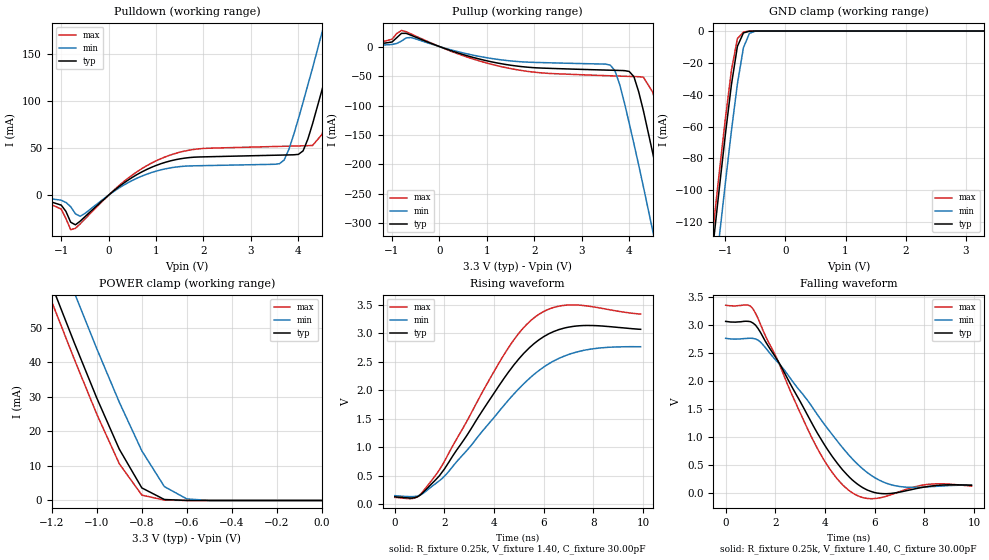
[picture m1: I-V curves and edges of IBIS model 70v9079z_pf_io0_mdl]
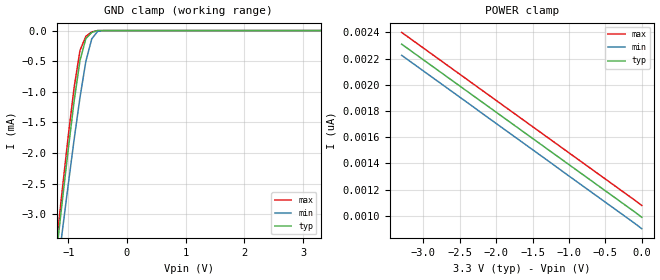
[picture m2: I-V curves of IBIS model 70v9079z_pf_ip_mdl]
| IBIS file 70v9079p.ibs created by s2ibis2 version 1.0
| North Carolina State University Electronics Research Laboratory  1995
[IBIS ver]   2.1
[File name]   70v9079p.ibs
[File Rev]   2.0
[Date]   06/15/97
[Source]   Integrated Device Technology, Inc.
[Notes]   1.Temperatures: typ=25C, min=100C, max=0C 2.Cemos8_5v process.
   3.RRmp rates based on 50 ohm load.
[Disclaimer]   This information is for modeling purpose only, and is not
   guaranteed.
[Copyright]   Copyright 1997, Integrated Device Technology, Inc. all rights
   reserved
|   Component 70v9079p
[Component]   70v9079p
[Manufacturer]   Integrated Device Technology
[Package]
| variable   typ   min   max
R_pkg   100.00m   90.00m   0.11
L_pkg   4.50nH   3.50nH   5.50nH
C_pkg   0.72pF   0.62pF   0.82pF
[Pin]  signal_name   model_name   R_pin   L_pin   C_pin
1   NC   NC
2   NC   NC
3   A7L   70v9079z_pf_ip_mdl
4   A8L   70v9079z_pf_ip_mdl
5   A19L   70v9079z_pf_ip_mdl
6   A10L   70v9079z_pf_ip_mdl
7   A11L   70v9079z_pf_ip_mdl
8   A12L   70v9079z_pf_ip_mdl
9   A13L   70v9079z_pf_ip_mdl
10   A14L   70v9079z_pf_ip_mdl
11   NC   NC
12   NC   NC
13   VCC   POWER
14   NC   NC
15   NC   NC
16   NC   NC
17   NC   NC
18   CE0BL   70v9079z_pf_ip_mdl
19   CE1L   70v9079z_pf_ip_mdl
20   CNTRSTBL   70v9079z_pf_ip_mdl
21   RWBL   70v9079z_pf_ip_mdl
22   OEBL   70v9079z_pf_ip_mdl
23   VCC   POWER
24   NC   NC
25   NC   NC
26   GND   GND
27   NC   NC
28   IO7L   70v9079z_pf_io0_mdl
29   IO6L   70v9079z_pf_io0_mdl
30   IO5L   70v9079z_pf_io0_mdl
31   IO4L   70v9079z_pf_io0_mdl
32   IO3L   70v9079z_pf_io0_mdl
33   IO2L   70v9079z_pf_io0_mdl
34   GND   GND
35   IO1L   70v9079z_pf_io0_mdl
36   IO0L   70v9079z_pf_io0_mdl
37   VCC   POWER
38   GND   GND
39   IO0R   70v9079z_pf_io0_mdl
40   IO1R   70v9079z_pf_io0_mdl
41   IO2R   70v9079z_pf_io0_mdl
42   VCC   POWER
43   IO3R   70v9079z_pf_io0_mdl
44   IO4R   70v9079z_pf_io0_mdl
45   IO5R   70v9079z_pf_io0_mdl
46   IO6R   70v9079z_pf_io0_mdl
47   IO7R   70v9079z_pf_io0_mdl
48   NC   NC
49   NC   NC
50   NC   NC
51   NC   NC
52   GND   GND
53   FT/PIPEBR   70v9079z_pf_ip_mdl
54   OEBR   70v9079z_pf_ip_mdl
55   RWBR   70v9079z_pf_ip_mdl
56   CNTRSTBR   70v9079z_pf_ip_mdl
57   CE1R   70v9079z_pf_ip_mdl
58   CE0BR   70v9079z_pf_ip_mdl
59   NC   NC
60   NC   NC
61   NC   NC
62   NC   NC
63   GND   GND
64   NC   NC
65   NC   NC
66   A14R   70v9079z_pf_ip_mdl
67   A13R   70v9079z_pf_ip_mdl
68   A12R   70v9079z_pf_ip_mdl
69   A11R   70v9079z_pf_ip_mdl
70   A10R   70v9079z_pf_ip_mdl
71   A9R   70v9079z_pf_ip_mdl
72   A8R   70v9079z_pf_ip_mdl
73   A7R   70v9079z_pf_ip_mdl
74   NC   NC
75   NC   NC
76   NC   NC
77   NC   NC
78   A6R   70v9079z_pf_ip_mdl
79   A5R   70v9079z_pf_ip_mdl
80   A4R   70v9079z_pf_ip_mdl
81   A3R   70v9079z_pf_ip_mdl
82   A2R   70v9079z_pf_ip_mdl
83   A1R   70v9079z_pf_ip_mdl
84   A0R   70v9079z_pf_ip_mdl
85   CNTENBR   70v9079z_pf_ip_mdl
86   CLKR   70v9079z_pf_ip_mdl
87   ADSBR   70v9079z_pf_ip_mdl
88   GND   GND
89   ADSBL   70v9079z_pf_ip_mdl
90   CLKL   70v9079z_pf_ip_mdl
91   CNTENBL   70v9079z_pf_ip_mdl
92   A0L   70v9079z_pf_ip_mdl
93   A1L   70v9079z_pf_ip_mdl
94   A2L   70v9079z_pf_ip_mdl
95   A3L   70v9079z_pf_ip_mdl
96   A4L   70v9079z_pf_ip_mdl
97   A5L   70v9079z_pf_ip_mdl
98   A6L   70v9079z_pf_ip_mdl
99   NC   NC
100   NC   NC
| Models and submodels in the file (2): 70v9079z_pf_io0_mdl (I/O), 70v9079z_pf_ip_mdl (Input)
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| in0  in0   dummy_model
| oel0 oel0   dummy_model
| in1  in1   dummy_model
| oel1 oel1   dummy_model
| in2  in2   dummy_model
| oel2 oel2   dummy_model
|   Model 70v9079z_pf_io0_mdl
[Model]   70v9079z_pf_io0_mdl
Model_type   I/O
Polarity   Non-Inverting
Enable   Active-High
Vinl =  0.800V
Vinh =  2.000V
Vmeas =  1.500V
C_comp   3.00pF   NA   NA
[Temperature Range]   25.00   100.00   0.000
[Voltage Range]   3.30V   3.00V   3.60V
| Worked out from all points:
|   slope of the pulldown table from 0 to 0.495 V, typ, clamps not added: 26.4 ohm
|   slope of the pullup table from 0 to 0.495 V, typ, clamps not added: 36.7 ohm
|   GND clamp passes 1 mA (typ) near -0.68 V on its own axis
|   POWER clamp passes 1 mA (typ) near -0.72 V on its own axis
|   rising waveform, R_fixture 0.25k, V_fixture 1.40, C_fixture 30.00pF: 20-80 % time 2.72ns typ, 3.16ns min, 2.49ns max; typ from 0.129 V to 3.07 V
|   falling waveform, R_fixture 0.25k, V_fixture 1.40, C_fixture 30.00pF: 20-80 % time 2.25ns typ, 2.7ns min, 2.02ns max; typ from 3.06 V to 0.143 V
[Pulldown]
| voltage   I(typ)   I(min)   I(max)
-3.3V     200uA      -200uA     300uA
-1.5V     -2.6mA     -2mA       -3.2mA
-1V       -10.54mA   -5.35mA    -14.74mA
-800mV    -28.71mA   -12.22mA   -36.61mA
-600mV    -27.58mA   -22.43mA   -30.49mA
1.2V      34.94mA    27.97mA    40.73mA
3.6V      42.47mA    33.33mA    51.74mA
4.1V      47.03mA    98.69mA    52.36mA
4.5V      112mA      173mA      64.64mA
4.9V      189mA      250mA      136mA
5.1V      228mA      289mA      175mA
6.6V      528mA      581mA      475mA
[Pullup]
| voltage   I(typ)   I(min)   I(max)
-3.3V     800uA      700uA      800uA
-1.5V     1.7mA      1.2mA      1.9mA
-800mV    22.41mA    9.33mA     27.36mA
1.4V      -30.42mA   -23.5mA    -35.74mA
3.6V      -40.1mA    -31.4mA    -49.57mA
4V        -42.16mA   -130mA     -50.61mA
4.2V      -76.73mA   -201mA     -51.13mA
4.5V      -182mA     -314mA     -77.89mA
4.9V      -334mA     -467mA     -220mA
5.1V      -411mA     -545mA     -296mA
5.3V      -490mA     -623mA     -374mA
6.6V      -1.02A     -1.149A    -901mA
[GND_clamp]
| voltage   I(typ)   I(min)   I(max)
-3.3V     -926mA     -959mA     -917mA
-1.3V     -168mA     -199mA     -158mA
-1.2V     -133mA     -164mA     -123mA
-1.1V     -98.42mA   -129mA     -88.29mA
-1V       -64.89mA   -95.35mA   -54.96mA
-900mV    -33.82mA   -62.85mA   -24.8mA
-800mV    -9.641mA   -33.21mA   -4.754mA
-700mV    -1.198mA   -10.52mA   -651uA
-600mV    -120uA     -1.465mA   -37.42uA
-500mV    -204nA     -55uA      -25.38nA
3.3V      2.97nA     32.7nA     2.341nA
[POWER_clamp]
| voltage   I(typ)   I(min)   I(max)
-3.3V     435mA      448mA      431mA
-1.2V     62.3mA     76.81mA    57.54mA
-1.1V     45.66mA    60.16mA    40.9mA
-1V       29.64mA    43.91mA    24.98mA
-900mV    14.84mA    28.42mA    10.64mA
-800mV    3.64mA     14.36mA    1.558mA
-700mV    287uA      4.021mA    111uA
-600mV    11.81uA    442uA      364nA
-500mV    64.91nA    16.3uA     9.871nA
0V        2.981nA    2.733nA    3.257nA
[Ramp]
| variable   typ   min   max
dV/dt_r   0.98/2.70n   0.76/2.97n   1.16/2.55n
dV/dt_f   1.12/2.47n   0.90/2.94n   1.32/2.17n
R_load = 50.00
[Rising Waveform]
R_fixture = 0.25k
V_fixture = 1.40
C_fixture = 30.00pF
R_dut = 100.00m
L_dut = 4.50nH
C_dut = 0.72pF
| time   V(typ)   V(min)   V(max)
0s        129mV      149mV      119mV
900ps     126mV      140mV      127mV
1.5ns     365mV      315mV      426mV
2.1ns     686mV      538mV      835mV
4.5ns     2.271V     1.788V     2.695V
5.1ns     2.602V     2.073V     3.056V
5.7ns     2.85V      2.311V     3.303V
6.4ns     3.031V     2.514V     3.454V
7.2ns     3.122V     2.656V     3.498V
9.9ns     3.07V      2.764V     3.337V
[Falling Waveform]
R_fixture = 0.25k
V_fixture = 1.40
C_fixture = 30.00pF
R_dut = 100.00m
L_dut = 4.50nH
C_dut = 0.72pF
| time   V(typ)   V(min)   V(max)
0s        3.058V     2.757V     3.346V
1.1ns     3.029V     2.756V     3.281V
2.3ns     2.202V     2.229V     2.148V
3.7ns     1.067V     1.397V     794mV
4.4ns     592mV      984mV      309mV
5ns       281mV      662mV      40.92mV
5.9ns     27.05mV    309mV      -94.97mV
6.8ns     6.943mV    138mV      -2.288mV
8.2ns     125mV      117mV      162mV
9.9ns     143mV      149mV      129mV
|   Model 70v9079z_pf_ip_mdl
[Model]   70v9079z_pf_ip_mdl
Model_type   Input
Vinl =  0.800V
Vinh =  2.000V
Vmeas =  1.500V
C_comp   3.00pF   NA   NA
[Temperature Range]   25.00   100.00   0.000
[Voltage Range]   3.30V   3.00V   3.60V
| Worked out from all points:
|   GND clamp passes 1 mA (typ) near -0.88 V on its own axis
[GND_clamp]
| voltage   I(typ)   I(min)   I(max)
-3.3V     -22.75mA   -21.12mA   -23.35mA
-1.2V     -3.629mA   -4.041mA   -3.47mA
-1.1V     -2.771mA   -3.268mA   -2.581mA
-1V       -1.937mA   -2.511mA   -1.721mA
-900mV    -1.151mA   -1.778mA   -927uA
-800mV    -487uA     -1.09mA    -323uA
-700mV    -130uA     -501uA     -93.54uA
-600mV    -31.23uA   -136uA     -21.92uA
-500mV    -23.28nA   -13.02uA   -2.254nA
-400mV    -898pA     -216nA     -544pA
3.3V      990pA      1.023nA    960pA
[POWER_clamp]
| voltage   I(typ)   I(min)   I(max)
-3.3V     2.31nA     2.225nA    2.4nA
-2.3V     1.91nA     1.825nA    2nA
-100mV    1.03nA     943pA      1.12nA
0V        988pA      901pA      1.078nA
